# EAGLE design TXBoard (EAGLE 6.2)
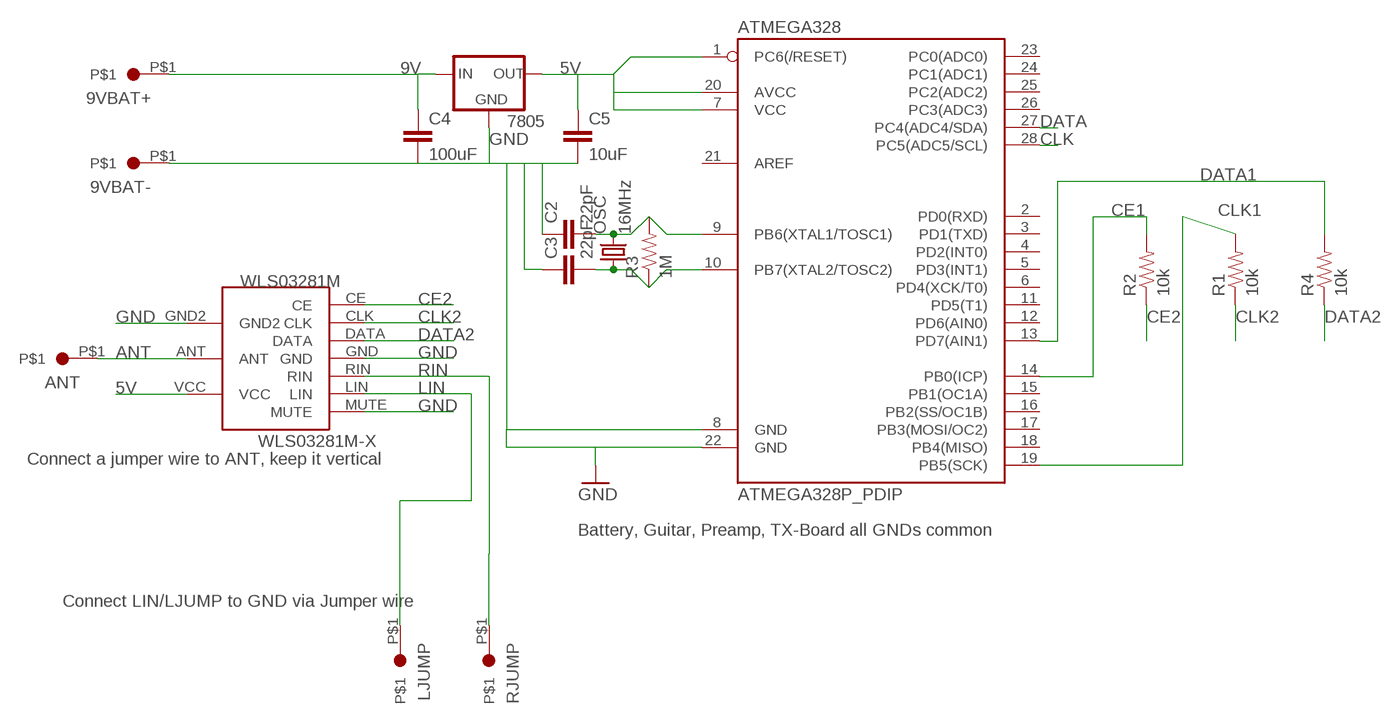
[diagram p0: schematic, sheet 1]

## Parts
9VBAT+  JUMPERDOT  [JUMPERDOT]
9VBAT-  JUMPERDOT  [JUMPERDOT]
7805  V_REG_78XXSIDE  [78XXL]
ANT  JUMPERDOT  [JUMPERDOT]
ATMEGA328  ATMEGA328P_PDIP  [DIL28-3]
C2  22pF  CAPPTH  [CAP-PTH-SMALL]
C3  22pF  CAPPTH  [CAP-PTH-SMALL]
C4  100uF  CAPPTH  [CAP-PTH-SMALL]
C5  10uF  CAPPTH  [CAP-PTH-SMALL]
LJUMP  JUMPERDOT  [JUMPERDOT]
OSC  16MHz  CRYSTALHC18U-V  [HC18U-V]
R1  10k  RESISTORAXIAL-0.3  [AXIAL-0.3]
R2  10k  RESISTORAXIAL-0.3  [AXIAL-0.3]
R3  1M  RESISTORAXIAL-0.3  [AXIAL-0.3]
R4  10k  RESISTORAXIAL-0.3  [AXIAL-0.3]
RJUMP  JUMPERDOT  [JUMPERDOT]
WLS03281M  WLS03281M-X  [WLS..PCB_TX]

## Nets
5V: 7805.OUT ATMEGA328.1(PC6(/RESET)) ATMEGA328.7(VCC) ATMEGA328.20(AVCC) C5.1 WLS03281M.VCC
9V: 9VBAT+.P$1 7805.IN C4.1
ANT: ANT.P$1 WLS03281M.ANT
CE1: ATMEGA328.14(PB0(ICP)) R2.P$2
CE2: R2.P$1 WLS03281M.CE
CLK: ATMEGA328.28(PC5(ADC5/SCL))
CLK1: ATMEGA328.19(PB5(SCK)) R1.P$2
CLK2: R1.P$1 WLS03281M.CLK
DATA: ATMEGA328.27(PC4(ADC4/SDA))
DATA1: ATMEGA328.13(PD7(AIN1)) R4.P$2
DATA2: R4.P$1 WLS03281M.DATA
GND: 9VBAT-.P$1 7805.GND ATMEGA328.8(GND) ATMEGA328.22(GND) C2.1 C3.1 C4.2 C5.2 WLS03281M.GND WLS03281M.GND2 WLS03281M.MUTE
LIN: LJUMP.P$1 WLS03281M.LIN
N$1: ATMEGA328.9(PB6(XTAL1/TOSC1)) C2.2 OSC.2 R3.P$2
N$2: ATMEGA328.10(PB7(XTAL2/TOSC2)) C3.2 OSC.1 R3.P$1
RIN: RJUMP.P$1 WLS03281M.RIN
Unconnected: ATMEGA328.2(PD0(RXD)) ATMEGA328.3(PD1(TXD)) ATMEGA328.4(PD2(INT0)) ATMEGA328.5(PD3(INT1)) ATMEGA328.6(PD4(XCK/T0)) ATMEGA328.11(PD5(T1)) ATMEGA328.12(PD6(AIN0)) ATMEGA328.15(PB1(OC1A)) ATMEGA328.16(PB2(SS/OC1B)) ATMEGA328.17(PB3(MOSI/OC2)) ATMEGA328.18(PB4(MISO)) ATMEGA328.21(AREF) ATMEGA328.23(PC0(ADC0)) ATMEGA328.24(PC1(ADC1)) ATMEGA328.25(PC2(ADC2)) ATMEGA328.26(PC3(ADC3))

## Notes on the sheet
- Connect a jumper wire to ANT, keep it vertical
- Battery, Guitar, Preamp, TX-Board all GNDs common
- Connect LIN/LJUMP to GND via Jumper wire

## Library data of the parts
9VBAT+ 9VBAT- ANT LJUMP RJUMP = fz:JUMPERDOT
7805 = SparkFun-PowerIC:V_REG_78XX: Voltage Regulator Standard 7805 5V regulator. IGO (Input Ground Output). Spark Fun Electronics SKU : COM-00107
ATMEGA328 = SparkFun-DigitalIC:ATMEGA328P_PDIP: uC used in the Arduino 32kb flash, 1k EEPROM, 2k SRAM This is the through-hole version of this chip.
C2-C5 = SparkFun-Passives:CAP: Capacitor
OSC = crystal:CRYSTAL: CRYSTAL; OC_FARNELL: unknown; OC_NEWARK: unknown
R1-R4 = SparkFun-Passives:RESISTOR: Resistor
WLS03281M = fz:WLS03281M

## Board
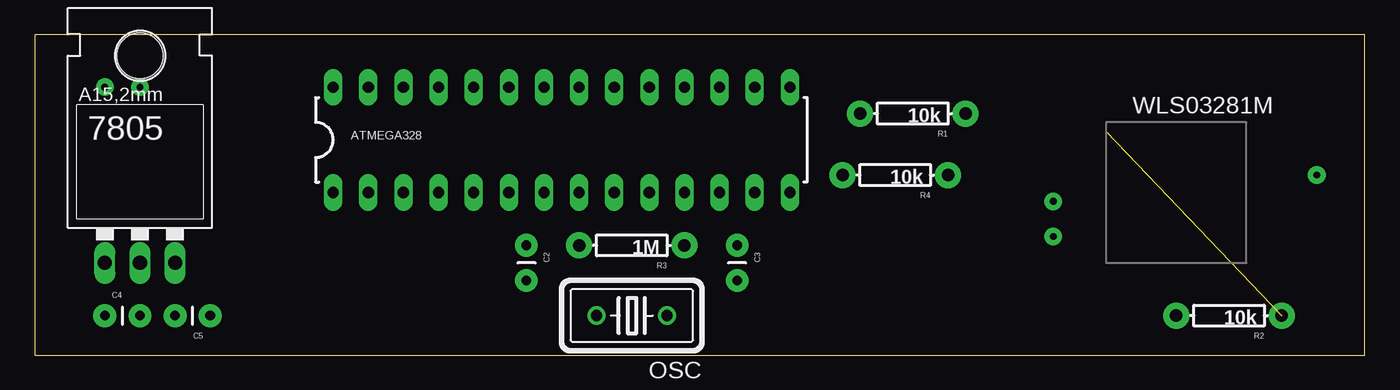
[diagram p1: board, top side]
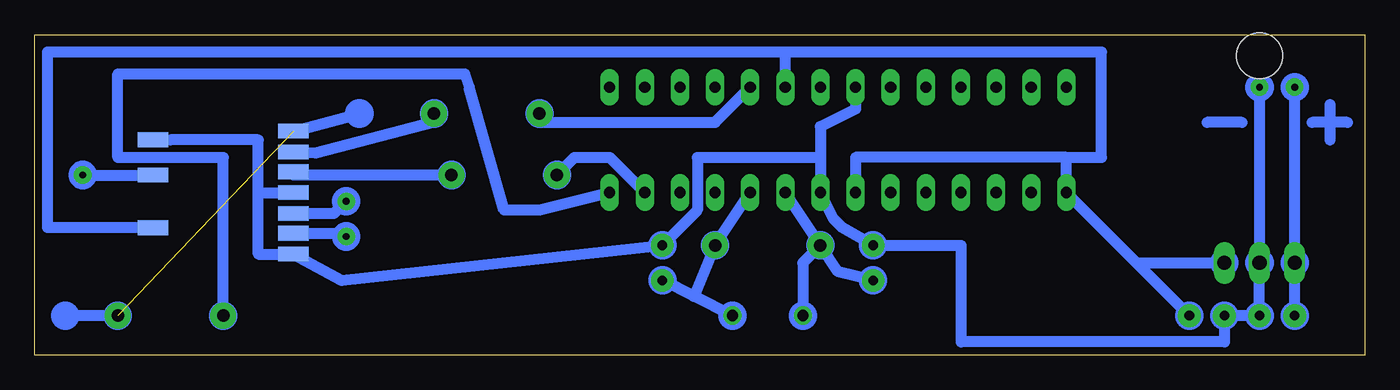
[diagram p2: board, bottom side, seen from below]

Size 96.19 x 23.17 mm. Coordinates in mm from the lower left corner, seen from the top.
Outline: 0,0 96.19,0 96.19,23.17 0,23.17 0,0
Copper layers (1*16): Top 0.035mm / dielectric 1.5mm / Bottom 0.035mm
Design rules: minimum track width 10mil, minimum drill 24mil, track to track 8mil, track to pad 8mil, pad to pad 8mil, via to via 8mil, smd to smd 8mil, copper to edge 40mil, drill to drill 8mil, minimum pad ring 10mil, minimum via ring 8mil, stop-mask expansion 4mil, vias tented up to drill 0mil, thermal gap 10mil

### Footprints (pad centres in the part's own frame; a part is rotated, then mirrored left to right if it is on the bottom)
JUMPERDOT = drill 0.5 pad 1.27: P$1 0,0
78XXL = drill 1.016 long: GND 0,-3.81; IN -2.54,-3.81; OUT 2.54,-3.81 | hole 3.302: 0,11.176
DIL28-3 = drill 0.813 long: 1 -16.51,-3.81; 2 -13.97,-3.81; 3 -11.43,-3.81; 4 -8.89,-3.81; 5 -6.35,-3.81; 6 -3.81,-3.81; 7 -1.27,-3.81; 8 1.27,-3.81; 9 3.81,-3.81; 10 6.35,-3.81; 11 8.89,-3.81; 12 11.43,-3.81; 13 13.97,-3.81; 14 16.51,-3.81; 15 16.51,3.81; 16 13.97,3.81; 17 11.43,3.81; 18 8.89,3.81; 19 6.35,3.81; 20 3.81,3.81; 21 1.27,3.81; 22 -1.27,3.81; 23 -3.81,3.81; 24 -6.35,3.81; 25 -8.89,3.81; 26 -11.43,3.81; 27 -13.97,3.81; 28 -16.51,3.81
CAP-PTH-SMALL = drill 0.7 pad 1.651: 1 0,0; 2 2.54,0
HC18U-V = drill 0.813: 1 -2.54,0; 2 2.54,0
AXIAL-0.3 = drill 0.9 pad 1.88: P$1 -3.81,0; P$2 3.81,0
WLS..PCB_TX = smd 2.184 x 1.067 bottom: ANT 10.16,6.35; CE 0,9.525; CLK 0,8.017; DATA 0,6.588; GND 0,5.08; GND2 10.16,8.89; LIN 0,2.143; MUTE 0,0.635; RIN 0,3.572; VCC 10.16,2.54

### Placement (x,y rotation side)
9VBAT+  5.08,19.37 0 top
9VBAT-  7.62,19.37 0 top
7805  7.62,10.48 0 top
ANT  92.71,13.02 0 top
ATMEGA328  38.1,15.56 0 top
C2  35.56,7.94 270 top
C3  50.8,7.94 270 top
C4  5.08,2.86 0 top
C5  12.7,2.86 180 top
LJUMP  73.66,8.57 0 top
OSC  43.18,2.86 180 top
R1  63.5,17.46 180 top
R2  86.36,2.86 180 top
R3  43.18,7.94 180 top
R4  62.23,13.02 180 top
RJUMP  73.66,11.11 0 top
WLS03281M  77.47,6.67 0 top

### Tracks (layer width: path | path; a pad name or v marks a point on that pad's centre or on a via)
5V
  Bottom 0.813: C5.1 16.51,6.67 | 16.51,6.67 ATMEGA328.1 21.59,14.29 | 16.51,6.67 7805.OUT | 41.91,21.91 95.25,21.91 95.25,9.21 WLS03281M.VCC | 21.59,14.29 36.83,14.29 ATMEGA328.7 36.83,13.02 | ATMEGA328.20 41.91,21.91 | 21.59,14.29 19.05,14.29 19.05,21.91 41.91,21.91
9V
  Bottom 0.813: C4.1 7805.IN 9VBAT+.P$1
ANT
  Bottom 0.813: ANT.P$1 WLS03281M.ANT
CE1
  Bottom 0.813: R2.P$2 82.55,14.29 90.17,14.29 90.17,20.32 65.09,20.32 64.77,19.37 62.23,10.48 59.69,10.48 ATMEGA328.14
CE2  (1 unrouted)
  Bottom 0.813: WLS03281M.CE 72.71,17.46 | R2.P$1 93.98,2.86
CLK1
  Bottom 0.813: ATMEGA328.19 46.99,16.83 59.69,16.83 R1.P$2
CLK2
  Bottom 0.254: 77.47,14.29 WLS03281M.CLK
  Bottom 0.813: R1.P$1 67.31,16.83 75.88,14.6 WLS03281M.CLK
DATA1
  Bottom 0.813: ATMEGA328.13 54.61,14.29 57.15,14.29 R4.P$2
DATA2
  Bottom 0.813: R4.P$1 77.47,13.02 WLS03281M.DATA
GND
  Bottom 0.254: WLS03281M.GND2 86.36,15.56
  Bottom 0.813: 80.01,11.75 WLS03281M.GND | 80.01,11.75 80.01,7.3 WLS03281M.MUTE 73.98,5.4 C3.1 48.26,10.48 48.26,14.29 39.37,14.29 | 9VBAT-.P$1 7805.GND C4.2 C5.2 10.16,0.95 29.21,0.95 29.21,7.94 C2.1 37.78,9.21 38.42,9.84 ATMEGA328.8 39.37,14.29 | ATMEGA328.22 36.83,17.78 39.37,16.51 39.37,14.29 | 80.01,11.75 80.01,15.56 86.36,15.56
LIN
  Bottom 0.254: 77.47,9.21 WLS03281M.LIN
  Bottom 0.406: 73.9,8.81 LJUMP.P$1
  Bottom 0.813: WLS03281M.LIN 73.9,8.81
N$1
  Bottom 0.813: OSC.2 40.64,6.67 R3.P$2 | C2.2 38.1,6.03 R3.P$2 | R3.P$2 ATMEGA328.9
N$2
  Bottom 0.813: ATMEGA328.10 R3.P$1 48.51,4.25 | OSC.1 48.51,4.25 | 48.51,4.25 C3.2
N$5
  Bottom 0.813: 2.54,18.1 2.54,15.56
N$6
  Bottom 0.813: 1.27,16.83 3.81,16.83
N$7
  Bottom 0.813: 8.89,16.83 11.43,16.83
RIN
  Bottom 0.254: 77.47,10.48 WLS03281M.RIN
  Bottom 0.813: WLS03281M.RIN 74.53,10.24 RJUMP.P$1
(copper drawn outside any net)
  shapes: Bottom circle x28

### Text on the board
tDocu: Ajmp | Ajmp

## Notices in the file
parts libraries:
SparkFun-DigitalIC: Licensing: CC v3.0 Share-Alike You are welcome to use this library for commercial purposes.
